PROGRAM MAIN_FAST
(* This task handles position data between drives and CNC *)
(* Its rate must be identical to the rate of CNC-TASK-GEO! *)
VAR
	iAxis			: USINT;	(* counter for the axis number *)
END_VAR

(* --------------------------------------------- *)
(* Triamec Motion AG, 6340 Baar, Switzerland     *)
(* Sample Code may be adapted to customer need   *)
(* --------------------------------------------- *)

(* Sync the trialink *)
gTrialink.CallFast();

FOR iAxis := 1 TO N_AXES DO
	(* get the coordinates from the NC and write it to the drive *)
	gAxes[iAxis].fastPositionCmd := gCncAxes[iAxis].CallFastPosCmd();
	gAxes[iAxis].CallFast( Trialink := gTrialink );

	(* get the actual position from the drive and pass it to NC *)
	gCncAxes[iAxis].CallFastPosAct(gAxes[iAxis].ActualPositionFast(Trialink := gTrialink));
END_FOR

publish1.CallFast(Trialink := gTrialink);

END_PROGRAM
